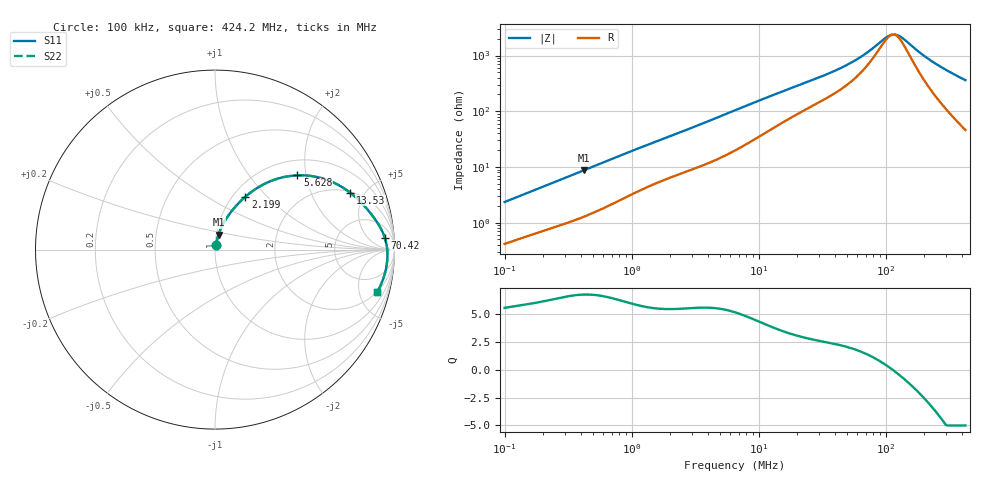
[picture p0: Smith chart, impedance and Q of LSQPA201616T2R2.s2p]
! LSQPA201616T2R2  S-PARAMETER MODEL  ( General Type )
! Model Generated by TAIYO YUDEN Corporation (http://www.ty-top.com)
! Version 2.0
! TAIYO YUDEN Control No. 100810NF25SB-FKC
! Copyright(c) 2007 TAIYO YUDEN CO.,LTD. All Rights Reserved.
! Product Description (link to TY-COMPAS)
! https://ds.yuden.co.jp/TYCOMPAS/or/detail?pn=LSQPA201616T2R2M&u=M
! Products Name : Inductors
! Characteristics :
!  Inductance : 2.2 uH , SRF(min) : 70 MHz , DC Resistance(max) : 0.26 Ohm
!  Rated Current : Saturation :750 mA , Temp Rise : 720 mA (40 degC)
!  Case Size : 2.0 x 1.6 / 0.079 x 0.063 [mm/inch] , Thickness : 1.6 / 0.063 [mm/inch]
!  (Conditions: Temperature = 25 degC , DC Bias Current/Voltage = 0A / 0V)
! External Node Assignments :
!  1  o---GGG---o  2
! GND o---------o GND
! Frequency Range : 0.1MHz  -  424.248007MHz  [ 402 STEP ]
# MHz S RI R 50
! Freq[MHz].  S11 Real  S11 Imag  S21 Real  S21 Imag  S12 Real  S12 Imag  S22 Real  S22 Imag
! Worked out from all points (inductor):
!   401 points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, 100 kHz to 424.2 MHz, reference 50 ohm
!   read as one part in series: L = 3.6 uH near 104.3 kHz
!   highest Q = 6.76 at 422.4 kHz (marker M1), where L = 3.27 uH
!   self-resonance near 113.6 MHz
!   S11 on the Smith chart (normalised r, x): 100 kHz: 1.01, +0.05; 2.199 MHz: 1.14, +0.76; 5.628 MHz: 1.33, +1.78; 13.53 MHz: 2.05, +3.91; 70.42 MHz: 14, +18; 424.2 MHz: 1.92, -7.18
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0.1  0.00467 0.0229  0.9953 -0.0229  0.9953 -0.0229  0.00467 0.0229
0.40516  0.0189 0.0809  0.9811 -0.0809  0.9811 -0.0809  0.0189 0.0809
0.422439  0.0199 0.084  0.9801 -0.084  0.9801 -0.084  0.0199 0.084
0.895881  0.0544 0.1592  0.9456 -0.1592  0.9456 -0.1592  0.0544 0.1592
1.641544  0.1196 0.246  0.8804 -0.246  0.8804 -0.246  0.1196 0.246
2.19897  0.1697 0.2949  0.8303 -0.2949  0.8303 -0.2949  0.1697 0.2949
3.409333  0.2795 0.368  0.7205 -0.368  0.7205 -0.368  0.2795 0.368
5.627643  0.459 0.4138  0.541 -0.4138  0.541 -0.4138  0.459 0.4138
6.650878  0.5246 0.4115  0.4754 -0.4115  0.4754 -0.4115  0.5246 0.4115
9.685496  0.6599 0.3738  0.3401 -0.3738  0.3401 -0.3738  0.6599 0.3738
13.52778  0.7522 0.3179  0.2478 -0.3179  0.2478 -0.3179  0.7522 0.3179
26.38981  0.8646 0.2051  0.1354 -0.2051  0.1354 -0.2051  0.8646 0.2051
46.37678  0.9202 0.1244  0.0798 -0.1244  0.0798 -0.1244  0.9202 0.1244
58.35259  0.936 0.0926  0.064 -0.0926  0.064 -0.0926  0.936 0.0926
70.41765  0.9459 0.0667  0.0541 -0.0667  0.0541 -0.0667  0.9459 0.0667
106.9209  0.9588 0.0086  0.0412 -0.0086  0.0412 -0.0086  0.9588 0.0086
116.2355  0.9599 -0.00325  0.0401 0.00325  0.0401 0.00325  0.9599 -0.00325
129.028  0.9608 -0.0183  0.0392 0.0183  0.0392 0.0183  0.9608 -0.0183
187.9  0.9579 -0.076  0.0421 0.076  0.0421 0.076  0.9579 -0.076
231.5354  0.9517 -0.1118  0.0483 0.1118  0.0483 0.1118  0.9517 -0.1118
316.7037  0.9336 -0.1729  0.0664 0.1729  0.0664 0.1729  0.9336 -0.1729
424.248  0.9027 -0.239  0.0973 0.239  0.0973 0.239  0.9027 -0.239
